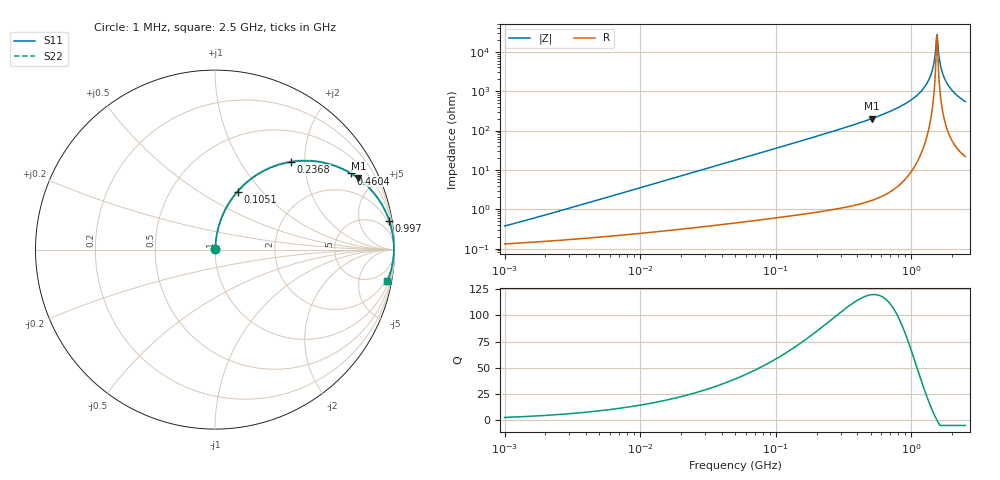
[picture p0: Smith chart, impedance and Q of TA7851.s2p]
# MHz S MA R 50
!Freq  MagS11  AngS11  MagS21  AngS21  MagS12  AngS12  MagS22  AngS22
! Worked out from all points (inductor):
!   801 points, 1 MHz to 2.5 GHz, reference 50 ohm
!   read as one part in series: L = 56 nH near 1.169 MHz
!   highest Q = 120 at 507.7 MHz (marker M1), where L = 62.8 nH
!   self-resonance near 1.533 GHz
!   S11 on the Smith chart (normalised r, x): 1 MHz: 1.00, +0.01; 105.1 MHz: 1.01, +0.74; 236.8 MHz: 1.02, +1.71; 460.4 MHz: 1.03, +3.56; 997 MHz: 1, +12; 2.5 GHz: 1, -11
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1  0.003753 69.2  0.9987 -0.2  0.9987 -0.2  0.003753 69.2
3.70813  0.01315 81.4  0.9981 -0.7  0.9981 -0.7  0.01315 81.4
13.61641  0.04781 84.0  0.9962 -2.7  0.9962 -2.7  0.04781 84.0
50  0.1727 78.6  0.9806 -9.9  0.9806 -9.9  0.1727 78.6
105.1415  0.3466 68.8  0.9323 -20.3  0.9323 -20.3  0.3466 68.8
185.4065  0.5489 56.0  0.8292 -33.3  0.8292 -33.3  0.5489 56.0
236.7612  0.6456 49.2  0.7567 -40.2  0.7567 -40.2  0.6456 49.2
460.4002  0.8685 29.2  0.4884 -60.3  0.4884 -60.3  0.8685 29.2
507.703  0.8918 26.4  0.4451 -63.1  0.4451 -63.1  0.8918 26.4
680.8203  0.9453 18.5  0.3178 -71.0  0.3178 -71.0  0.9453 18.5
996.9699  0.9841 9.4  0.1634 -79.7  0.1634 -79.7  0.9841 9.4
1177.303  0.9924 5.7  0.1001 -82.8  0.1001 -82.8  0.9924 5.7
1323.907  0.9955 3.2  0.05646 -83.9  0.05646 -83.9  0.9955 3.2
1417.716  0.9964 1.8  0.03129 -82.6  0.03129 -82.6  0.9964 1.8
1445.72  0.9966 1.4  0.02415 -81.2  0.02415 -81.2  0.9966 1.4
1503.398  0.9967 0.5  0.01012 -70.5  0.01012 -70.5  0.9967 0.5
1548.161  0.9966 -0.1  0.003616 19.4  0.003616 19.4  0.9966 -0.1
1594.257  0.9964 -0.7  0.01248 72.8  0.01248 72.8  0.9964 -0.7
1674.155  0.9958 -1.7  0.03016 81.1  0.03016 81.1  0.9958 -1.7
1810.402  0.994 -3.4  0.05888 82.5  0.05888 82.5  0.994 -3.4
2076.055  0.9887 -6.3  0.1097 80.9  0.1097 80.9  0.9887 -6.3
2500  0.9763 -10.4  0.1804 77.3  0.1804 77.3  0.9763 -10.4
